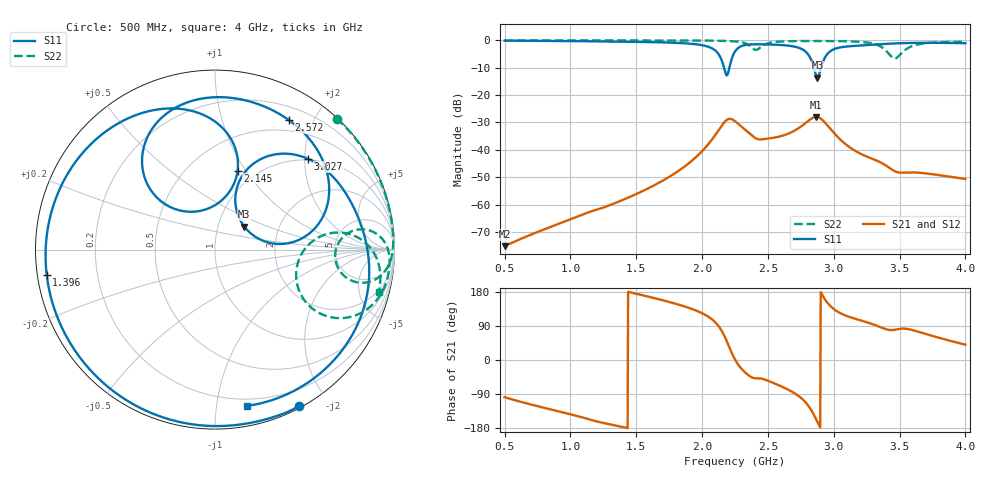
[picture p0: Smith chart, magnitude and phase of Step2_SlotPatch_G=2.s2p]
! TOUCHSTONE file generated by CST MICROWAVE STUDIO
! Date and time: Mon May 18 02:50:58 2020
! Project name: DualBand_DualMode_Antenna_FD_SteppedDesign.cst
! Parameters = {FPL=20; FPW=20; L=50; ST=10; SW=30; W=52; WF=7; ext=10; gap=1; inset=13}
! Header version: 2015
! Port assignment regex: !\s*Touchstone port\s*([0-9]+)\s*=\s*CST MWS port\s*([0-9]+)\s*\(\"(.*)\"\)(\s*mode\s*([0-9]+))?.*
! Touchstone port assignment:
! Touchstone port 1 = CST MWS port 1 ("")
! Touchstone port 2 = CST MWS port 2 ("")
# GHz S MA R 50
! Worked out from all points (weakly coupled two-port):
!   1006 points, 500 MHz to 4 GHz, reference 50 ohm
!   highest |S21| = -27.98 dB at 2.866 GHz (marker M1); lowest = -75.2 dB at 500 MHz (marker M2)
!   lowest |S11| = -13.7 dB at 2.877 GHz (marker M3), VSWR 1.52, Z = 66.8 + j17.9 ohm
!   |S11| at or under -10 dB: 2.167 GHz to 2.207 GHz (40.22 MHz wide, 1.84 % of centre); 2.849 GHz to 2.903 GHz (53.96 MHz wide, 1.88 % of centre)
!   |S22| runs from -6.6 to 0.0 dB; largest |S21 - S12| = 4.8e-05
!   S11 on the Smith chart (normalised r, x): 500 MHz: 0.02, -1.67; 1.396 GHz: 0.03, -0.07; 2.145 GHz: 0.82, +0.92; 2.572 GHz: 0.36, +1.66; 3.027 GHz: 0.97, +2.07; 4 GHz: 0.15, -1.21
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0.5  0.9886 -61.8  0.0001737 -98.2  0.0001737 -98.2  0.9974 47.0
0.7905  0.9816 -97.5  0.0003446 -125.4  0.0003445 -125.3  0.998 28.6
1.0845  0.9671 -133.6  0.0006462 -150.8  0.000639 -149.8  0.9979 18.6
1.396  0.9481 -171.5  0.001211 -176.8  0.001212 -176.2  0.9972 11.5
1.669  0.9247 154.3  0.002477 160.6  0.002476 160.5  0.996 6.6
1.9875  0.8277 108.2  0.00882 125.6  0.008819 125.6  0.9919 0.9
2.145  0.4583 74.1  0.02684 79.3  0.02684 79.3  0.9827 -2.8
2.1905  0.2311 111.1  0.03558 47.1  0.03558 47.1  0.9757 -4.3
2.25  0.6277 130.3  0.03347 1.3  0.03347 1.3  0.9595 -6.7
2.362  0.8421 96.7  0.01992 -42.6  0.01992 -42.6  0.7988 -12.9
2.453  0.8491 79.6  0.01557 -49.3  0.01557 -49.3  0.7803 7.8
2.572  0.831 60.4  0.01716 -65.1  0.01716 -65.1  0.9459 2.5
2.7435  0.7202 27.9  0.02591 -97.7  0.02591 -97.7  0.9741 -3.2
2.8345  0.4081 5.0  0.03765 -135.4  0.03765 -135.4  0.9753 -5.5
2.866  0.2284 20.1  0.03992 -156.3  0.03992 -156.3  0.9751 -6.3
2.8765  0.2077 38.0  0.03973 -163.7  0.03973 -163.7  0.9751 -6.5
2.9465  0.5453 64.6  0.02896 153.6  0.02896 153.6  0.9749 -8.3
3.027  0.7242 44.3  0.01747 128.1  0.01747 128.1  0.9718 -10.7
3.265  0.8257 9.3  0.007304 98.1  0.007284 98.1  0.9063 -21.8
3.419  0.8706 -9.3  0.00476 79.6  0.004777 79.9  0.5665 -29.2
3.5485  0.8948 -25.2  0.00385 82.5  0.003851 82.6  0.6867 8.0
4  0.8887 -78.6  0.002943 40.4  0.002943 40.4  0.9426 -14.4
